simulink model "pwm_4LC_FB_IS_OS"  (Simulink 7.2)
settings: Solver=ode3  SolverMode=SingleTasking  StartTime=0.0  StopTime=0.1  FixedStep=10e-6  MaxStep=1e-4  RelTol=1e-3

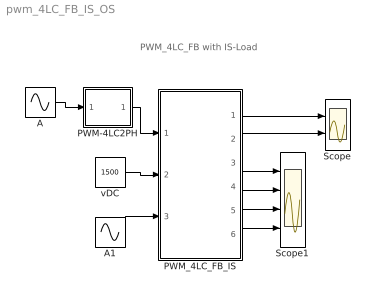
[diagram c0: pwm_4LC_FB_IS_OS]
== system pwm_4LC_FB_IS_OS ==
  note: PWM_4LC_FB with IS-Load
  A : Sin  Amplitude=.8  Frequency=2*pi*50  Phase=[0]  SampleTime=0
  A1 : Sin  Amplitude=500  Frequency=2*pi*50  Phase=[0 ]  SampleTime=0
  PWM-4LC2PH : Subsystem  mask(PWM-4LC1PH){FT=500, PHT1=0, PHT2=-120, PHT3=-240, DT=1e-6}
      mask prompts: FT "Frequency of Trian Sig."; PHT1 "Phase Angle of 1st Trian. Sig."; PHT2 "Phase Angle of 2nd Trian. Sig."; PHT3 "Phase Angle of 3rd Trian. Sig."; DT "Dead Time"
      mask help: Pulse Width Modulation for 1 Phase 4 Level Floating Capacitor Converter
  PWM_4LC_FB_IS : Subsystem  mask(pwm_4LC_FB_IS_OS){C1=10e-3, VC10=2*1500/3, C2=10e-3, VC20=1500/3}
      mask prompts: C1 "Cap C1"; VC10 "Initial Cap Voltage VC10"; C2 "Cap C2"; VC20 "Initial Cap Voltage VC20"
      mask help: Open Source 4-Level FC PWM FB Converter with IS load Input Vector u: u[0]= TD1.gate u[1]= TD2.gate u[2]= TD3.gate u[3]= TD4.gate u[4]= TD5.gate u[5]= TD6.gate u[6]= TD7.gate u[7]= TD8.gate u[8]= TD9.gate u[9]= TD10.gate u[10]= TD11.gate u[11]= TD12.gate u[12]= VDC u[13]= IA, Load Current as AC Current source Output Vector y: y[0]= Va.v, Output AC Voltage to middle point y[1]= Ia.I, Output AC Current y[2]= T1.I y[3]= D1.I y[4]= T1.V y[5]= T2.I y[6]= D2.I y[7]= T2.V y[8]= T3.I y[9]= D3.I y[10]= T3.V y[11]= IDC1, Input DC Current y[12]= IDC2, Input DC Current Parameter Vector p: p[0]= C1 p[1]= VC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
  Scope : Scope  NumInputPorts=2
  Scope1 : Scope  NumInputPorts=4
  vDC : Constant  Value=1500  OutDataType=sfix(16)  OutScaling=2^0
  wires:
  A/1 -> PWM-4LC2PH/1(In1)
  PWM-4LC2PH/1(Out1) -> PWM_4LC_FB_IS/1(Sw)
  PWM_4LC_FB_IS/1(vA) -> Scope/1
  PWM_4LC_FB_IS/2(iA) -> Scope/2
  vDC/1 -> PWM_4LC_FB_IS/2(vDC)
  A1/1 -> PWM_4LC_FB_IS/3(i_A)
  PWM_4LC_FB_IS/3(iT1,iD1,vT1) -> Scope1/1
  PWM_4LC_FB_IS/4(iT2,ID2,vT2) -> Scope1/2
  PWM_4LC_FB_IS/5(iT3,iD3,vT3) -> Scope1/3
  PWM_4LC_FB_IS/6(iDC1,IDC2) -> Scope1/4

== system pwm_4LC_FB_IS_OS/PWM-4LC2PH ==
  In1 : Inport  OutDataType=sfix(16)  OutScaling=2^0
  Gain : Gain  Gain=-1  ParameterDataType=sfix(16)  ParameterScaling=2^0  OutDataType=sfix(16)  OutScaling=2^0
  Mux : Mux  Inputs=2
  PWM-4LC1PH : Subsystem  mask(PWM-4LC1PH){FT=900, PHT1=0, PHT2=-120, PHT3=-240, DT=1e-6}
      mask prompts: FT "Frequency of Trian Sig."; PHT1 "Phase Angle of 1st Trian. Sig."; PHT2 "Phase Angle of 2nd Trian. Sig."; PHT3 "Phase Angle of 3rd Trian. Sig."; DT "Dead Time"
      mask help: Pulse Width Modulation for 1 Phase 4 Level Floating Capacitor Converter
  PWM-4LC1PH1 : Subsystem  mask(PWM-4LC1PH){FT=900, PHT1=0, PHT2=-120, PHT3=-240, DT=1e-6}
      mask prompts: FT "Frequency of Trian Sig."; PHT1 "Phase Angle of 1st Trian. Sig."; PHT2 "Phase Angle of 2nd Trian. Sig."; PHT3 "Phase Angle of 3rd Trian. Sig."; DT "Dead Time"
      mask help: Pulse Width Modulation for 1 Phase 4 Level Floating Capacitor Converter
  Out1 : Outport
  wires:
  In1/1 -> PWM-4LC1PH/1(In1), Gain/1
  PWM-4LC1PH1/1(Out1) -> Mux/2
  PWM-4LC1PH/1(Out1) -> Mux/1
  Mux/1 -> Out1/1
  Gain/1 -> PWM-4LC1PH1/1(In1)

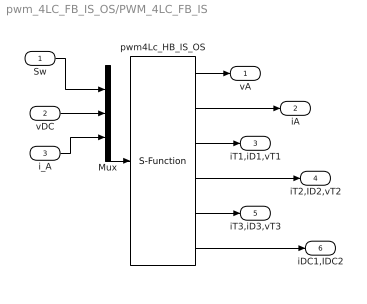
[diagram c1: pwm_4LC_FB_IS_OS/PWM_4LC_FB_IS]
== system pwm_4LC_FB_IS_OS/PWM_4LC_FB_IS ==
  Sw : Inport  OutDataType=sfix(16)  OutScaling=2^0
  vDC : Inport  Port=2  OutDataType=sfix(16)  OutScaling=2^0
  i_A : Inport  Port=3  OutDataType=sfix(16)  OutScaling=2^0
  Mux : Mux  Inputs="[12  1  1]"
  pwm4Lc_HB_IS_OS : S-Function  FunctionName=s_pwm_4LC_FB_IS_OS  Parameters="[C1  VC10  C2  VC20]"  EnableBusSupport=off
  vA : Outport  OutDataType=sfix(16)  OutScaling=2^0
  iA : Outport  Port=2  OutDataType=sfix(16)  OutScaling=2^0
  iT1,iD1,vT1 : Outport  Port=3  OutDataType=sfix(16)  OutScaling=2^0
  iT2,ID2,vT2 : Outport  Port=4  OutDataType=sfix(16)  OutScaling=2^0
  iT3,iD3,vT3 : Outport  Port=5  OutDataType=sfix(16)  OutScaling=2^0
  iDC1,IDC2 : Outport  Port=6  OutDataType=sfix(16)  OutScaling=2^0
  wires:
  pwm4Lc_HB_IS_OS/6 -> iDC1,IDC2/1
  pwm4Lc_HB_IS_OS/2 -> iA/1
  pwm4Lc_HB_IS_OS/1 -> vA/1
  i_A/1 -> Mux/3
  Mux/1 -> pwm4Lc_HB_IS_OS/1
  vDC/1 -> Mux/2
  Sw/1 -> Mux/1
  pwm4Lc_HB_IS_OS/3 -> iT1,iD1,vT1/1
  pwm4Lc_HB_IS_OS/4 -> iT2,ID2,vT2/1
  pwm4Lc_HB_IS_OS/5 -> iT3,iD3,vT3/1

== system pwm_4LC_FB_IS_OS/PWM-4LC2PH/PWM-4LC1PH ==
  In1 : Inport  OutDataType=sfix(16)  OutScaling=2^0
  Mux : Mux  Inputs=6
  PWM-2L-1PH : Subsystem  mask(PWM-2L-1PH){FT=FT, PHT=PHT1, DT=DT}
      mask prompts: FT "Triangular Frequency"; PHT "Trian. Phase Angle (Degree)"; DT "Dead Time"
      mask help: Pulse Width Modulation for 1 Phase Converter
  PWM-2L-1PH1 : Subsystem  mask(PWM-2L-1PH){FT=FT, PHT=PHT2, DT=DT}
      mask prompts: FT "Triangular Frequency"; PHT "Trian. Phase Angle (Degree)"; DT "Dead Time"
      mask help: Pulse Width Modulation for 1 Phase Converter
  PWM-2L-1PH2 : Subsystem  mask(PWM-2L-1PH){FT=FT, PHT=PHT3, DT=DT}
      mask prompts: FT "Triangular Frequency"; PHT "Trian. Phase Angle (Degree)"; DT "Dead Time"
      mask help: Pulse Width Modulation for 1 Phase Converter
  Out1 : Outport
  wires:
  PWM-2L-1PH/1(Out1) -> Mux/1
  PWM-2L-1PH1/1(Out1) -> Mux/2
  PWM-2L-1PH1/2(Out2) -> Mux/5
  PWM-2L-1PH2/1(Out1) -> Mux/3
  PWM-2L-1PH2/2(Out2) -> Mux/4
  Mux/1 -> Out1/1
  In1/1 -> PWM-2L-1PH/1(In1), PWM-2L-1PH1/1(In1), PWM-2L-1PH2/1(In1)
  PWM-2L-1PH/2(Out2) -> Mux/6

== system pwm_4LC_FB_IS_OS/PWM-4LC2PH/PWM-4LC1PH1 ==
  In1 : Inport  OutDataType=sfix(16)  OutScaling=2^0
  Mux : Mux  Inputs=6
  PWM-2L-1PH : Subsystem  mask(PWM-2L-1PH){FT=FT, PHT=PHT1, DT=DT}
      mask prompts: FT "Triangular Frequency"; PHT "Trian. Phase Angle (Degree)"; DT "Dead Time"
      mask help: Pulse Width Modulation for 1 Phase Converter
  PWM-2L-1PH1 : Subsystem  mask(PWM-2L-1PH){FT=FT, PHT=PHT2, DT=DT}
      mask prompts: FT "Triangular Frequency"; PHT "Trian. Phase Angle (Degree)"; DT "Dead Time"
      mask help: Pulse Width Modulation for 1 Phase Converter
  PWM-2L-1PH2 : Subsystem  mask(PWM-2L-1PH){FT=FT, PHT=PHT3, DT=DT}
      mask prompts: FT "Triangular Frequency"; PHT "Trian. Phase Angle (Degree)"; DT "Dead Time"
      mask help: Pulse Width Modulation for 1 Phase Converter
  Out1 : Outport
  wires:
  PWM-2L-1PH/2(Out2) -> Mux/6
  In1/1 -> PWM-2L-1PH2/1(In1), PWM-2L-1PH1/1(In1), PWM-2L-1PH/1(In1)
  Mux/1 -> Out1/1
  PWM-2L-1PH2/2(Out2) -> Mux/4
  PWM-2L-1PH2/1(Out1) -> Mux/3
  PWM-2L-1PH1/2(Out2) -> Mux/5
  PWM-2L-1PH1/1(Out1) -> Mux/2
  PWM-2L-1PH/1(Out1) -> Mux/1

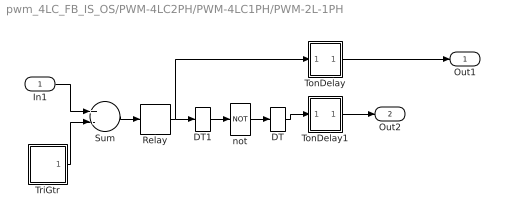
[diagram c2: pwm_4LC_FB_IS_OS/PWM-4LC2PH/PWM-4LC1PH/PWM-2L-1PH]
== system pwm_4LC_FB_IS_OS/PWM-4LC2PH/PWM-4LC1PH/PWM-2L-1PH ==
  In1 : Inport  OutDataType=sfix(16)  OutScaling=2^0
  DT : DataTypeConversion
  DT1 : DataTypeConversion
  Relay : Relay  OutDataType=sfix(16)  OutScaling=2^0
  Sum : Sum  Inputs=+-  OutDataType=sfix(16)  OutScaling=2^0
  TonDelay : Subsystem  mask(TonDelay){DT=DT}
      mask prompts: DT "Dead Time"
      mask help: Turn on dead time to protect against short circuit of the converter leg
  TonDelay1 : Subsystem  mask(TonDelay){DT=DT}
      mask prompts: DT "Dead Time"
      mask help: Turn on dead time to protect against short circuit of the converter leg
  TriGtr : Subsystem  mask(TriGtr){T=1/FT, Td=PHT/FT/360}
      mask prompts: T "Period Time"; Td "Time Delay"
      mask help: Triangular Wave Generator with variable time delay
  not : Logic  Operator=NOT  Inputs=1
  Out1 : Outport  InitialOutput=0
  Out2 : Outport  Port=2  InitialOutput=0
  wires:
  DT1/1 -> not/1
  DT/1 -> TonDelay1/1(s1)
  In1/1 -> Sum/1
  TriGtr/1(O) -> Sum/2
  Sum/1 -> Relay/1
  not/1 -> DT/1
  TonDelay1/1(s1d) -> Out2/1
  Relay/1 -> DT1/1, TonDelay/1(s1)
  TonDelay/1(s1d) -> Out1/1

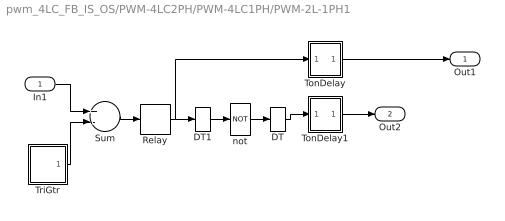
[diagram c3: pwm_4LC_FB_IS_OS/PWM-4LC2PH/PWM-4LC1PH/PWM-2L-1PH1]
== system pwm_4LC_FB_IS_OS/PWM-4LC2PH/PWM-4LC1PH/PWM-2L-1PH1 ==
  In1 : Inport  OutDataType=sfix(16)  OutScaling=2^0
  DT : DataTypeConversion
  DT1 : DataTypeConversion
  Relay : Relay  OutDataType=sfix(16)  OutScaling=2^0
  Sum : Sum  Inputs=+-  OutDataType=sfix(16)  OutScaling=2^0
  TonDelay : Subsystem  mask(TonDelay){DT=DT}
      mask prompts: DT "Dead Time"
      mask help: Turn on dead time to protect against short circuit of the converter leg
  TonDelay1 : Subsystem  mask(TonDelay){DT=DT}
      mask prompts: DT "Dead Time"
      mask help: Turn on dead time to protect against short circuit of the converter leg
  TriGtr : Subsystem  mask(TriGtr){T=1/FT, Td=PHT/FT/360}
      mask prompts: T "Period Time"; Td "Time Delay"
      mask help: Triangular Wave Generator with variable time delay
  not : Logic  Operator=NOT  Inputs=1
  Out1 : Outport  InitialOutput=0
  Out2 : Outport  Port=2  InitialOutput=0
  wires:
  TonDelay/1(s1d) -> Out1/1
  Relay/1 -> TonDelay/1(s1), DT1/1
  TonDelay1/1(s1d) -> Out2/1
  not/1 -> DT/1
  Sum/1 -> Relay/1
  TriGtr/1(O) -> Sum/2
  In1/1 -> Sum/1
  DT/1 -> TonDelay1/1(s1)
  DT1/1 -> not/1

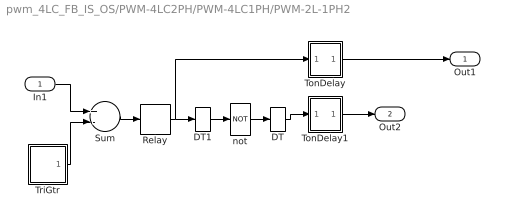
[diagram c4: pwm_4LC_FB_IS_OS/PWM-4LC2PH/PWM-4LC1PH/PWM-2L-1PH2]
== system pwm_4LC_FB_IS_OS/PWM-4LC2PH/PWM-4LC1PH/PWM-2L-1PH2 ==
  In1 : Inport  OutDataType=sfix(16)  OutScaling=2^0
  DT : DataTypeConversion
  DT1 : DataTypeConversion
  Relay : Relay  OutDataType=sfix(16)  OutScaling=2^0
  Sum : Sum  Inputs=+-  OutDataType=sfix(16)  OutScaling=2^0
  TonDelay : Subsystem  mask(TonDelay){DT=DT}
      mask prompts: DT "Dead Time"
      mask help: Turn on dead time to protect against short circuit of the converter leg
  TonDelay1 : Subsystem  mask(TonDelay){DT=DT}
      mask prompts: DT "Dead Time"
      mask help: Turn on dead time to protect against short circuit of the converter leg
  TriGtr : Subsystem  mask(TriGtr){T=1/FT, Td=PHT/FT/360}
      mask prompts: T "Period Time"; Td "Time Delay"
      mask help: Triangular Wave Generator with variable time delay
  not : Logic  Operator=NOT  Inputs=1
  Out1 : Outport  InitialOutput=0
  Out2 : Outport  Port=2  InitialOutput=0
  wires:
  DT1/1 -> not/1
  DT/1 -> TonDelay1/1(s1)
  In1/1 -> Sum/1
  TriGtr/1(O) -> Sum/2
  Sum/1 -> Relay/1
  not/1 -> DT/1
  TonDelay1/1(s1d) -> Out2/1
  Relay/1 -> DT1/1, TonDelay/1(s1)
  TonDelay/1(s1d) -> Out1/1

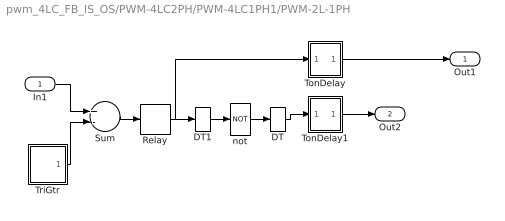
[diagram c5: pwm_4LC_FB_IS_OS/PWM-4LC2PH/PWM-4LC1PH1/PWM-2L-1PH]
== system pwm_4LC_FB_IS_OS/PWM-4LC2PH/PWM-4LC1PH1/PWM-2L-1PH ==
  In1 : Inport  OutDataType=sfix(16)  OutScaling=2^0
  DT : DataTypeConversion
  DT1 : DataTypeConversion
  Relay : Relay  OutDataType=sfix(16)  OutScaling=2^0
  Sum : Sum  Inputs=+-  OutDataType=sfix(16)  OutScaling=2^0
  TonDelay : Subsystem  mask(TonDelay){DT=DT}
      mask prompts: DT "Dead Time"
      mask help: Turn on dead time to protect against short circuit of the converter leg
  TonDelay1 : Subsystem  mask(TonDelay){DT=DT}
      mask prompts: DT "Dead Time"
      mask help: Turn on dead time to protect against short circuit of the converter leg
  TriGtr : Subsystem  mask(TriGtr){T=1/FT, Td=PHT/FT/360}
      mask prompts: T "Period Time"; Td "Time Delay"
      mask help: Triangular Wave Generator with variable time delay
  not : Logic  Operator=NOT  Inputs=1
  Out1 : Outport  InitialOutput=0
  Out2 : Outport  Port=2  InitialOutput=0
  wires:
  TonDelay/1(s1d) -> Out1/1
  Relay/1 -> TonDelay/1(s1), DT1/1
  TonDelay1/1(s1d) -> Out2/1
  not/1 -> DT/1
  Sum/1 -> Relay/1
  TriGtr/1(O) -> Sum/2
  In1/1 -> Sum/1
  DT/1 -> TonDelay1/1(s1)
  DT1/1 -> not/1

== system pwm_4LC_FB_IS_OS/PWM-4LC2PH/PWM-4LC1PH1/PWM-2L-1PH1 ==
  In1 : Inport  OutDataType=sfix(16)  OutScaling=2^0
  DT : DataTypeConversion
  DT1 : DataTypeConversion
  Relay : Relay  OutDataType=sfix(16)  OutScaling=2^0
  Sum : Sum  Inputs=+-  OutDataType=sfix(16)  OutScaling=2^0
  TonDelay : Subsystem  mask(TonDelay){DT=DT}
      mask prompts: DT "Dead Time"
      mask help: Turn on dead time to protect against short circuit of the converter leg
  TonDelay1 : Subsystem  mask(TonDelay){DT=DT}
      mask prompts: DT "Dead Time"
      mask help: Turn on dead time to protect against short circuit of the converter leg
  TriGtr : Subsystem  mask(TriGtr){T=1/FT, Td=PHT/FT/360}
      mask prompts: T "Period Time"; Td "Time Delay"
      mask help: Triangular Wave Generator with variable time delay
  not : Logic  Operator=NOT  Inputs=1
  Out1 : Outport  InitialOutput=0
  Out2 : Outport  Port=2  InitialOutput=0
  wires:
  DT1/1 -> not/1
  DT/1 -> TonDelay1/1(s1)
  In1/1 -> Sum/1
  TriGtr/1(O) -> Sum/2
  Sum/1 -> Relay/1
  not/1 -> DT/1
  TonDelay1/1(s1d) -> Out2/1
  Relay/1 -> DT1/1, TonDelay/1(s1)
  TonDelay/1(s1d) -> Out1/1

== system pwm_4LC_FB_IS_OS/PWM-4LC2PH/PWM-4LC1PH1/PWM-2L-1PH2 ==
  In1 : Inport  OutDataType=sfix(16)  OutScaling=2^0
  DT : DataTypeConversion
  DT1 : DataTypeConversion
  Relay : Relay  OutDataType=sfix(16)  OutScaling=2^0
  Sum : Sum  Inputs=+-  OutDataType=sfix(16)  OutScaling=2^0
  TonDelay : Subsystem  mask(TonDelay){DT=DT}
      mask prompts: DT "Dead Time"
      mask help: Turn on dead time to protect against short circuit of the converter leg
  TonDelay1 : Subsystem  mask(TonDelay){DT=DT}
      mask prompts: DT "Dead Time"
      mask help: Turn on dead time to protect against short circuit of the converter leg
  TriGtr : Subsystem  mask(TriGtr){T=1/FT, Td=PHT/FT/360}
      mask prompts: T "Period Time"; Td "Time Delay"
      mask help: Triangular Wave Generator with variable time delay
  not : Logic  Operator=NOT  Inputs=1
  Out1 : Outport  InitialOutput=0
  Out2 : Outport  Port=2  InitialOutput=0
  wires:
  TonDelay/1(s1d) -> Out1/1
  Relay/1 -> TonDelay/1(s1), DT1/1
  TonDelay1/1(s1d) -> Out2/1
  not/1 -> DT/1
  Sum/1 -> Relay/1
  TriGtr/1(O) -> Sum/2
  In1/1 -> Sum/1
  DT/1 -> TonDelay1/1(s1)
  DT1/1 -> not/1

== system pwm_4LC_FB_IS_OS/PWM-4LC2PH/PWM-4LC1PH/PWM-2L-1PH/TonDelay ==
  s1 : Inport  Orientation=down  OutDataType=sfix(16)  OutScaling=2^0
  Int : Integrator  ExternalReset=falling
  Rel1 : Relay  OnSwitchValue=DT  OutDataType=sfix(16)  OutScaling=2^0
  s1d : Outport  InitialOutput=0
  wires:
  Int/1 -> Rel1/1
  s1/1 -> Int/2, Int/1
  Rel1/1 -> s1d/1

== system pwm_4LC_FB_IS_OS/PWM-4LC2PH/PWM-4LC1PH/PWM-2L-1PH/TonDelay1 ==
  s1 : Inport  Orientation=down  OutDataType=sfix(16)  OutScaling=2^0
  Int : Integrator  ExternalReset=falling
  Rel1 : Relay  OnSwitchValue=DT  OutDataType=sfix(16)  OutScaling=2^0
  s1d : Outport  InitialOutput=0
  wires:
  Int/1 -> Rel1/1
  s1/1 -> Int/2, Int/1
  Rel1/1 -> s1d/1

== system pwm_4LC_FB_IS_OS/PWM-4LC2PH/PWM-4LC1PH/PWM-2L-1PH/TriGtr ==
  Clock : Clock
  S1 : Subsystem
  Sum : Sum  OutDataType=sfix(16)  OutScaling=2^0
  T : Constant  Value=T  OutDataType=sfix(16)  OutScaling=2^0
  Td : Constant  Value=Td  OutDataType=sfix(16)  OutScaling=2^0
  mod : Math  Operator=mod
  O : Outport  InitialOutput=0
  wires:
  mod/1 -> S1/1(In1)
  S1/1(Out1) -> O/1
  Clock/1 -> Sum/1
  T/1 -> mod/2
  Sum/1 -> mod/1
  Td/1 -> Sum/2

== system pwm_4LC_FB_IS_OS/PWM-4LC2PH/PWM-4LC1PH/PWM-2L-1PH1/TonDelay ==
  s1 : Inport  Orientation=down  OutDataType=sfix(16)  OutScaling=2^0
  Int : Integrator  ExternalReset=falling
  Rel1 : Relay  OnSwitchValue=DT  OutDataType=sfix(16)  OutScaling=2^0
  s1d : Outport  InitialOutput=0
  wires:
  Rel1/1 -> s1d/1
  s1/1 -> Int/1, Int/2
  Int/1 -> Rel1/1

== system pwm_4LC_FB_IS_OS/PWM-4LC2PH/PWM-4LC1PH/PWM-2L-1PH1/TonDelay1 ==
  s1 : Inport  Orientation=down  OutDataType=sfix(16)  OutScaling=2^0
  Int : Integrator  ExternalReset=falling
  Rel1 : Relay  OnSwitchValue=DT  OutDataType=sfix(16)  OutScaling=2^0
  s1d : Outport  InitialOutput=0
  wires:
  Rel1/1 -> s1d/1
  s1/1 -> Int/1, Int/2
  Int/1 -> Rel1/1

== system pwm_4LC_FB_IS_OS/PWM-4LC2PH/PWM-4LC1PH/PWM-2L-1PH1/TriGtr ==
  Clock : Clock
  S1 : Subsystem
  Sum : Sum  OutDataType=sfix(16)  OutScaling=2^0
  T : Constant  Value=T  OutDataType=sfix(16)  OutScaling=2^0
  Td : Constant  Value=Td  OutDataType=sfix(16)  OutScaling=2^0
  mod : Math  Operator=mod
  O : Outport  InitialOutput=0
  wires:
  Td/1 -> Sum/2
  Sum/1 -> mod/1
  T/1 -> mod/2
  Clock/1 -> Sum/1
  S1/1(Out1) -> O/1
  mod/1 -> S1/1(In1)

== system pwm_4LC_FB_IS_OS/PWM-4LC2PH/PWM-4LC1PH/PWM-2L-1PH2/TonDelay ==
  s1 : Inport  Orientation=down  OutDataType=sfix(16)  OutScaling=2^0
  Int : Integrator  ExternalReset=falling
  Rel1 : Relay  OnSwitchValue=DT  OutDataType=sfix(16)  OutScaling=2^0
  s1d : Outport  InitialOutput=0
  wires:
  Int/1 -> Rel1/1
  s1/1 -> Int/2, Int/1
  Rel1/1 -> s1d/1

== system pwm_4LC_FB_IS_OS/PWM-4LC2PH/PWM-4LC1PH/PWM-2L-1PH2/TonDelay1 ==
  s1 : Inport  Orientation=down  OutDataType=sfix(16)  OutScaling=2^0
  Int : Integrator  ExternalReset=falling
  Rel1 : Relay  OnSwitchValue=DT  OutDataType=sfix(16)  OutScaling=2^0
  s1d : Outport  InitialOutput=0
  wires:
  Int/1 -> Rel1/1
  s1/1 -> Int/2, Int/1
  Rel1/1 -> s1d/1

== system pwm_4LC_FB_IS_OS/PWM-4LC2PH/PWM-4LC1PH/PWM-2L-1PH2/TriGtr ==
  Clock : Clock
  S1 : Subsystem
  Sum : Sum  OutDataType=sfix(16)  OutScaling=2^0
  T : Constant  Value=T  OutDataType=sfix(16)  OutScaling=2^0
  Td : Constant  Value=Td  OutDataType=sfix(16)  OutScaling=2^0
  mod : Math  Operator=mod
  O : Outport  InitialOutput=0
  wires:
  mod/1 -> S1/1(In1)
  S1/1(Out1) -> O/1
  Clock/1 -> Sum/1
  T/1 -> mod/2
  Sum/1 -> mod/1
  Td/1 -> Sum/2

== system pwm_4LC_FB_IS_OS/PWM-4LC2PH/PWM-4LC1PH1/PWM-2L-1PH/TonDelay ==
  s1 : Inport  Orientation=down  OutDataType=sfix(16)  OutScaling=2^0
  Int : Integrator  ExternalReset=falling
  Rel1 : Relay  OnSwitchValue=DT  OutDataType=sfix(16)  OutScaling=2^0
  s1d : Outport  InitialOutput=0
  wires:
  Rel1/1 -> s1d/1
  s1/1 -> Int/1, Int/2
  Int/1 -> Rel1/1

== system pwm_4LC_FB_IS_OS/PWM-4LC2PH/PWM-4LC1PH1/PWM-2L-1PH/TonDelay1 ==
  s1 : Inport  Orientation=down  OutDataType=sfix(16)  OutScaling=2^0
  Int : Integrator  ExternalReset=falling
  Rel1 : Relay  OnSwitchValue=DT  OutDataType=sfix(16)  OutScaling=2^0
  s1d : Outport  InitialOutput=0
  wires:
  Rel1/1 -> s1d/1
  s1/1 -> Int/1, Int/2
  Int/1 -> Rel1/1

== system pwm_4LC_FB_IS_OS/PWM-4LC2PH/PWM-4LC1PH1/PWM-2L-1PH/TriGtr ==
  Clock : Clock
  S1 : Subsystem
  Sum : Sum  OutDataType=sfix(16)  OutScaling=2^0
  T : Constant  Value=T  OutDataType=sfix(16)  OutScaling=2^0
  Td : Constant  Value=Td  OutDataType=sfix(16)  OutScaling=2^0
  mod : Math  Operator=mod
  O : Outport  InitialOutput=0
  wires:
  Td/1 -> Sum/2
  Sum/1 -> mod/1
  T/1 -> mod/2
  Clock/1 -> Sum/1
  S1/1(Out1) -> O/1
  mod/1 -> S1/1(In1)

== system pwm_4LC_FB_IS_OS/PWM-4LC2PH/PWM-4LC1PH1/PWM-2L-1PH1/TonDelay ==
  s1 : Inport  Orientation=down  OutDataType=sfix(16)  OutScaling=2^0
  Int : Integrator  ExternalReset=falling
  Rel1 : Relay  OnSwitchValue=DT  OutDataType=sfix(16)  OutScaling=2^0
  s1d : Outport  InitialOutput=0
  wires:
  Int/1 -> Rel1/1
  s1/1 -> Int/2, Int/1
  Rel1/1 -> s1d/1

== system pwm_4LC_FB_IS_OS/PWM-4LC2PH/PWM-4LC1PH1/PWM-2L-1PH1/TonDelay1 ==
  s1 : Inport  Orientation=down  OutDataType=sfix(16)  OutScaling=2^0
  Int : Integrator  ExternalReset=falling
  Rel1 : Relay  OnSwitchValue=DT  OutDataType=sfix(16)  OutScaling=2^0
  s1d : Outport  InitialOutput=0
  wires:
  Int/1 -> Rel1/1
  s1/1 -> Int/2, Int/1
  Rel1/1 -> s1d/1

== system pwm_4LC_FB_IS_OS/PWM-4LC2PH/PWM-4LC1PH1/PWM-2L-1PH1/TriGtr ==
  Clock : Clock
  S1 : Subsystem
  Sum : Sum  OutDataType=sfix(16)  OutScaling=2^0
  T : Constant  Value=T  OutDataType=sfix(16)  OutScaling=2^0
  Td : Constant  Value=Td  OutDataType=sfix(16)  OutScaling=2^0
  mod : Math  Operator=mod
  O : Outport  InitialOutput=0
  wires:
  mod/1 -> S1/1(In1)
  S1/1(Out1) -> O/1
  Clock/1 -> Sum/1
  T/1 -> mod/2
  Sum/1 -> mod/1
  Td/1 -> Sum/2

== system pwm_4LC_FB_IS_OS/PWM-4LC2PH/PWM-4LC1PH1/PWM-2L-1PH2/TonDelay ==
  s1 : Inport  Orientation=down  OutDataType=sfix(16)  OutScaling=2^0
  Int : Integrator  ExternalReset=falling
  Rel1 : Relay  OnSwitchValue=DT  OutDataType=sfix(16)  OutScaling=2^0
  s1d : Outport  InitialOutput=0
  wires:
  Rel1/1 -> s1d/1
  s1/1 -> Int/1, Int/2
  Int/1 -> Rel1/1

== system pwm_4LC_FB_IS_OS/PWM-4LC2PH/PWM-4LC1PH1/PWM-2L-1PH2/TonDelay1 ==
  s1 : Inport  Orientation=down  OutDataType=sfix(16)  OutScaling=2^0
  Int : Integrator  ExternalReset=falling
  Rel1 : Relay  OnSwitchValue=DT  OutDataType=sfix(16)  OutScaling=2^0
  s1d : Outport  InitialOutput=0
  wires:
  Rel1/1 -> s1d/1
  s1/1 -> Int/1, Int/2
  Int/1 -> Rel1/1

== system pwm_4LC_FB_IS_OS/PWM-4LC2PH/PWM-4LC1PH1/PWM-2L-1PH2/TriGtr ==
  Clock : Clock
  S1 : Subsystem
  Sum : Sum  OutDataType=sfix(16)  OutScaling=2^0
  T : Constant  Value=T  OutDataType=sfix(16)  OutScaling=2^0
  Td : Constant  Value=Td  OutDataType=sfix(16)  OutScaling=2^0
  mod : Math  Operator=mod
  O : Outport  InitialOutput=0
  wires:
  Td/1 -> Sum/2
  Sum/1 -> mod/1
  T/1 -> mod/2
  Clock/1 -> Sum/1
  S1/1(Out1) -> O/1
  mod/1 -> S1/1(In1)

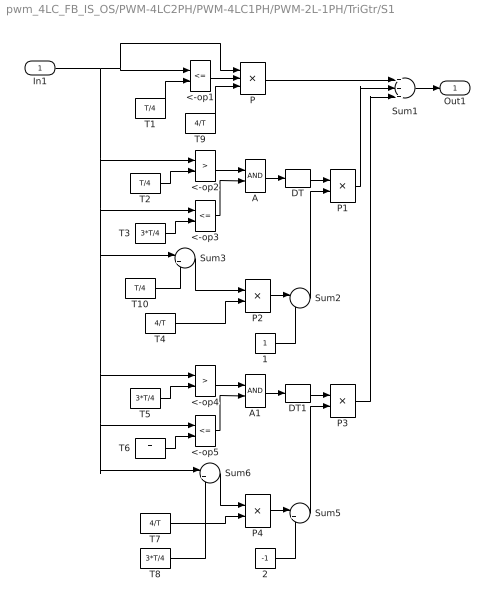
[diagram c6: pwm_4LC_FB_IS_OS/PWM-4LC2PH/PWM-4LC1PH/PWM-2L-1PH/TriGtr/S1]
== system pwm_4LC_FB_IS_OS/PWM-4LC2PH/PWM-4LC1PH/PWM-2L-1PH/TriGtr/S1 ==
  In1 : Inport  OutDataType=sfix(16)  OutScaling=2^0
  1 : Constant  OutDataType=sfix(16)  OutScaling=2^0
  2 : Constant  Value=-1  OutDataType=sfix(16)  OutScaling=2^0
  <-op1 : RelationalOperator  Operator=<=
  <-op2 : RelationalOperator  Operator=>
  <-op3 : RelationalOperator  Operator=<=
  <-op4 : RelationalOperator  Operator=>
  <-op5 : RelationalOperator  Operator=<=
  A : Logic  AllPortsSameDT=off
  A1 : Logic  AllPortsSameDT=off
  DT : DataTypeConversion
  DT1 : DataTypeConversion
  P : Product  Inputs=3  OutDataType=sfix(16)  OutScaling=2^0
  P{1..4} (4 alike) : Product  OutDataType=sfix(16)  OutScaling=2^0
  Sum1 : Sum  Inputs=+++  OutDataType=sfix(16)  OutScaling=2^0
  Sum2 : Sum  Inputs=|-+  OutDataType=sfix(16)  OutScaling=2^0
  Sum3 : Sum  Inputs=|+-  OutDataType=sfix(16)  OutScaling=2^0
  Sum5 : Sum  Inputs=|++  OutDataType=sfix(16)  OutScaling=2^0
  Sum6 : Sum  Inputs=|+-  OutDataType=sfix(16)  OutScaling=2^0
  T1 : Constant  Value=T/4  OutDataType=sfix(16)  OutScaling=2^0
  T10 : Constant  Value=T/4  OutDataType=sfix(16)  OutScaling=2^0
  T2 : Constant  Value=T/4  OutDataType=sfix(16)  OutScaling=2^0
  T3 : Constant  Value=3*T/4  OutDataType=sfix(16)  OutScaling=2^0
  T4 : Constant  Value=4/T  OutDataType=sfix(16)  OutScaling=2^0
  T5 : Constant  Value=3*T/4  OutDataType=sfix(16)  OutScaling=2^0
  T6 : Constant  Value=T  OutDataType=sfix(16)  OutScaling=2^0
  T7 : Constant  Value=4/T  OutDataType=sfix(16)  OutScaling=2^0
  T8 : Constant  Value=3*T/4  OutDataType=sfix(16)  OutScaling=2^0
  T9 : Constant  Value=4/T  OutDataType=sfix(16)  OutScaling=2^0
  Out1 : Outport
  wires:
  Sum1/1 -> Out1/1
  P3/1 -> Sum1/3
  T8/1 -> Sum6/2
  Sum5/1 -> P3/2
  2/1 -> Sum5/2
  P4/1 -> Sum5/1
  Sum6/1 -> P4/1
  T7/1 -> P4/2
  A1/1 -> DT1/1
  <-op5/1 -> A1/2
  T6/1 -> <-op5/2
  <-op4/1 -> A1/1
  T5/1 -> <-op4/2
  Sum2/1 -> P1/2
  1/1 -> Sum2/2
  P2/1 -> Sum2/1
  P1/1 -> Sum1/2
  In1/1 -> P/1, <-op1/1, Sum6/1, <-op5/1, <-op4/1, Sum3/1, <-op3/1, <-op2/1
  Sum3/1 -> P2/1
  T4/1 -> P2/2
  A/1 -> DT/1
  <-op3/1 -> A/2
  T3/1 -> <-op3/2
  <-op2/1 -> A/1
  T2/1 -> <-op2/2
  P/1 -> Sum1/1
  <-op1/1 -> P/2
  T1/1 -> <-op1/2
  DT/1 -> P1/1
  DT1/1 -> P3/1
  T9/1 -> P/3
  T10/1 -> Sum3/2

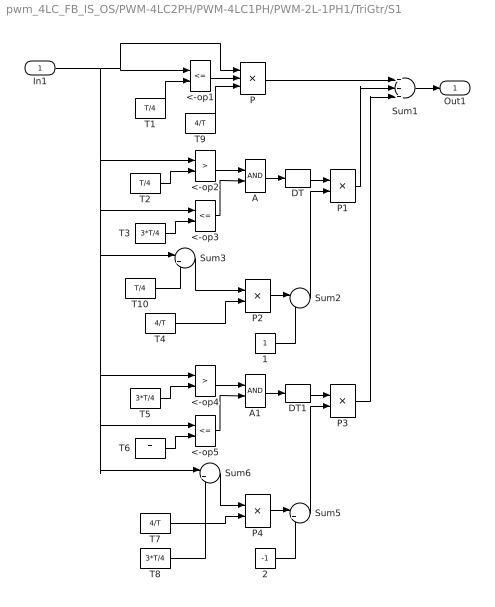
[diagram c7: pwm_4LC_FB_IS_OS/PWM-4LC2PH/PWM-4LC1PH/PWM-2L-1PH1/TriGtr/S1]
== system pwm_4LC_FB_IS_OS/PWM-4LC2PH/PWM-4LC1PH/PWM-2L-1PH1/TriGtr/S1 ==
  In1 : Inport  OutDataType=sfix(16)  OutScaling=2^0
  1 : Constant  OutDataType=sfix(16)  OutScaling=2^0
  2 : Constant  Value=-1  OutDataType=sfix(16)  OutScaling=2^0
  <-op1 : RelationalOperator  Operator=<=
  <-op2 : RelationalOperator  Operator=>
  <-op3 : RelationalOperator  Operator=<=
  <-op4 : RelationalOperator  Operator=>
  <-op5 : RelationalOperator  Operator=<=
  A : Logic  AllPortsSameDT=off
  A1 : Logic  AllPortsSameDT=off
  DT : DataTypeConversion
  DT1 : DataTypeConversion
  P : Product  Inputs=3  OutDataType=sfix(16)  OutScaling=2^0
  P{1..4} (4 alike) : Product  OutDataType=sfix(16)  OutScaling=2^0
  Sum1 : Sum  Inputs=+++  OutDataType=sfix(16)  OutScaling=2^0
  Sum2 : Sum  Inputs=|-+  OutDataType=sfix(16)  OutScaling=2^0
  Sum3 : Sum  Inputs=|+-  OutDataType=sfix(16)  OutScaling=2^0
  Sum5 : Sum  Inputs=|++  OutDataType=sfix(16)  OutScaling=2^0
  Sum6 : Sum  Inputs=|+-  OutDataType=sfix(16)  OutScaling=2^0
  T1 : Constant  Value=T/4  OutDataType=sfix(16)  OutScaling=2^0
  T10 : Constant  Value=T/4  OutDataType=sfix(16)  OutScaling=2^0
  T2 : Constant  Value=T/4  OutDataType=sfix(16)  OutScaling=2^0
  T3 : Constant  Value=3*T/4  OutDataType=sfix(16)  OutScaling=2^0
  T4 : Constant  Value=4/T  OutDataType=sfix(16)  OutScaling=2^0
  T5 : Constant  Value=3*T/4  OutDataType=sfix(16)  OutScaling=2^0
  T6 : Constant  Value=T  OutDataType=sfix(16)  OutScaling=2^0
  T7 : Constant  Value=4/T  OutDataType=sfix(16)  OutScaling=2^0
  T8 : Constant  Value=3*T/4  OutDataType=sfix(16)  OutScaling=2^0
  T9 : Constant  Value=4/T  OutDataType=sfix(16)  OutScaling=2^0
  Out1 : Outport
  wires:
  T10/1 -> Sum3/2
  T9/1 -> P/3
  DT1/1 -> P3/1
  DT/1 -> P1/1
  T1/1 -> <-op1/2
  <-op1/1 -> P/2
  P/1 -> Sum1/1
  T2/1 -> <-op2/2
  <-op2/1 -> A/1
  T3/1 -> <-op3/2
  <-op3/1 -> A/2
  A/1 -> DT/1
  T4/1 -> P2/2
  Sum3/1 -> P2/1
  In1/1 -> <-op2/1, <-op3/1, Sum3/1, <-op4/1, <-op5/1, Sum6/1, <-op1/1, P/1
  P1/1 -> Sum1/2
  P2/1 -> Sum2/1
  1/1 -> Sum2/2
  Sum2/1 -> P1/2
  T5/1 -> <-op4/2
  <-op4/1 -> A1/1
  T6/1 -> <-op5/2
  <-op5/1 -> A1/2
  A1/1 -> DT1/1
  T7/1 -> P4/2
  Sum6/1 -> P4/1
  P4/1 -> Sum5/1
  2/1 -> Sum5/2
  Sum5/1 -> P3/2
  T8/1 -> Sum6/2
  P3/1 -> Sum1/3
  Sum1/1 -> Out1/1

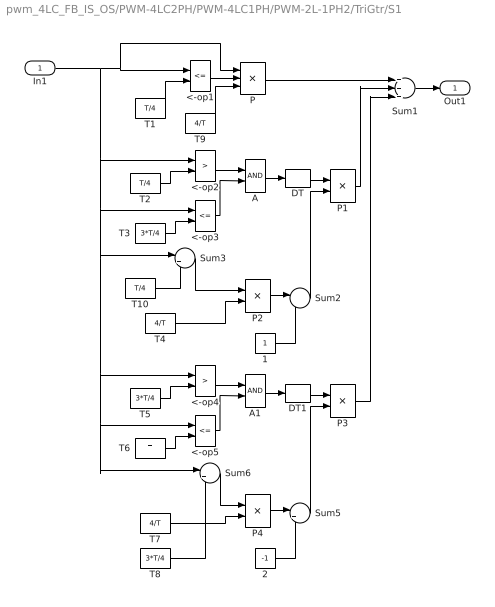
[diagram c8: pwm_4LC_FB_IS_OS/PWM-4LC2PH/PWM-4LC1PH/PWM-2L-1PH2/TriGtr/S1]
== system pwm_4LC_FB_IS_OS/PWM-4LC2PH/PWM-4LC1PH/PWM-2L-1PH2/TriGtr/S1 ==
  In1 : Inport  OutDataType=sfix(16)  OutScaling=2^0
  1 : Constant  OutDataType=sfix(16)  OutScaling=2^0
  2 : Constant  Value=-1  OutDataType=sfix(16)  OutScaling=2^0
  <-op1 : RelationalOperator  Operator=<=
  <-op2 : RelationalOperator  Operator=>
  <-op3 : RelationalOperator  Operator=<=
  <-op4 : RelationalOperator  Operator=>
  <-op5 : RelationalOperator  Operator=<=
  A : Logic  AllPortsSameDT=off
  A1 : Logic  AllPortsSameDT=off
  DT : DataTypeConversion
  DT1 : DataTypeConversion
  P : Product  Inputs=3  OutDataType=sfix(16)  OutScaling=2^0
  P{1..4} (4 alike) : Product  OutDataType=sfix(16)  OutScaling=2^0
  Sum1 : Sum  Inputs=+++  OutDataType=sfix(16)  OutScaling=2^0
  Sum2 : Sum  Inputs=|-+  OutDataType=sfix(16)  OutScaling=2^0
  Sum3 : Sum  Inputs=|+-  OutDataType=sfix(16)  OutScaling=2^0
  Sum5 : Sum  Inputs=|++  OutDataType=sfix(16)  OutScaling=2^0
  Sum6 : Sum  Inputs=|+-  OutDataType=sfix(16)  OutScaling=2^0
  T1 : Constant  Value=T/4  OutDataType=sfix(16)  OutScaling=2^0
  T10 : Constant  Value=T/4  OutDataType=sfix(16)  OutScaling=2^0
  T2 : Constant  Value=T/4  OutDataType=sfix(16)  OutScaling=2^0
  T3 : Constant  Value=3*T/4  OutDataType=sfix(16)  OutScaling=2^0
  T4 : Constant  Value=4/T  OutDataType=sfix(16)  OutScaling=2^0
  T5 : Constant  Value=3*T/4  OutDataType=sfix(16)  OutScaling=2^0
  T6 : Constant  Value=T  OutDataType=sfix(16)  OutScaling=2^0
  T7 : Constant  Value=4/T  OutDataType=sfix(16)  OutScaling=2^0
  T8 : Constant  Value=3*T/4  OutDataType=sfix(16)  OutScaling=2^0
  T9 : Constant  Value=4/T  OutDataType=sfix(16)  OutScaling=2^0
  Out1 : Outport
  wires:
  Sum1/1 -> Out1/1
  P3/1 -> Sum1/3
  T8/1 -> Sum6/2
  Sum5/1 -> P3/2
  2/1 -> Sum5/2
  P4/1 -> Sum5/1
  Sum6/1 -> P4/1
  T7/1 -> P4/2
  A1/1 -> DT1/1
  <-op5/1 -> A1/2
  T6/1 -> <-op5/2
  <-op4/1 -> A1/1
  T5/1 -> <-op4/2
  Sum2/1 -> P1/2
  1/1 -> Sum2/2
  P2/1 -> Sum2/1
  P1/1 -> Sum1/2
  In1/1 -> P/1, <-op1/1, Sum6/1, <-op5/1, <-op4/1, Sum3/1, <-op3/1, <-op2/1
  Sum3/1 -> P2/1
  T4/1 -> P2/2
  A/1 -> DT/1
  <-op3/1 -> A/2
  T3/1 -> <-op3/2
  <-op2/1 -> A/1
  T2/1 -> <-op2/2
  P/1 -> Sum1/1
  <-op1/1 -> P/2
  T1/1 -> <-op1/2
  DT/1 -> P1/1
  DT1/1 -> P3/1
  T9/1 -> P/3
  T10/1 -> Sum3/2

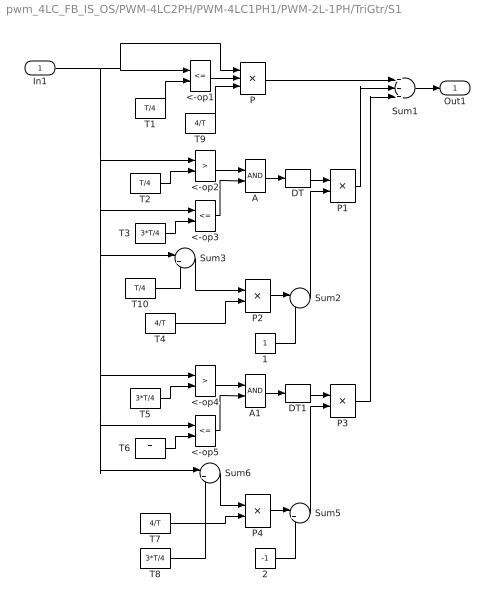
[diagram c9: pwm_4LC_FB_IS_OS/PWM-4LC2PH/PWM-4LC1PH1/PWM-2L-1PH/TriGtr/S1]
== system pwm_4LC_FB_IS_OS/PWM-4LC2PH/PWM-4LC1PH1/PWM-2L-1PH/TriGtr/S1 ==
  In1 : Inport  OutDataType=sfix(16)  OutScaling=2^0
  1 : Constant  OutDataType=sfix(16)  OutScaling=2^0
  2 : Constant  Value=-1  OutDataType=sfix(16)  OutScaling=2^0
  <-op1 : RelationalOperator  Operator=<=
  <-op2 : RelationalOperator  Operator=>
  <-op3 : RelationalOperator  Operator=<=
  <-op4 : RelationalOperator  Operator=>
  <-op5 : RelationalOperator  Operator=<=
  A : Logic  AllPortsSameDT=off
  A1 : Logic  AllPortsSameDT=off
  DT : DataTypeConversion
  DT1 : DataTypeConversion
  P : Product  Inputs=3  OutDataType=sfix(16)  OutScaling=2^0
  P{1..4} (4 alike) : Product  OutDataType=sfix(16)  OutScaling=2^0
  Sum1 : Sum  Inputs=+++  OutDataType=sfix(16)  OutScaling=2^0
  Sum2 : Sum  Inputs=|-+  OutDataType=sfix(16)  OutScaling=2^0
  Sum3 : Sum  Inputs=|+-  OutDataType=sfix(16)  OutScaling=2^0
  Sum5 : Sum  Inputs=|++  OutDataType=sfix(16)  OutScaling=2^0
  Sum6 : Sum  Inputs=|+-  OutDataType=sfix(16)  OutScaling=2^0
  T1 : Constant  Value=T/4  OutDataType=sfix(16)  OutScaling=2^0
  T10 : Constant  Value=T/4  OutDataType=sfix(16)  OutScaling=2^0
  T2 : Constant  Value=T/4  OutDataType=sfix(16)  OutScaling=2^0
  T3 : Constant  Value=3*T/4  OutDataType=sfix(16)  OutScaling=2^0
  T4 : Constant  Value=4/T  OutDataType=sfix(16)  OutScaling=2^0
  T5 : Constant  Value=3*T/4  OutDataType=sfix(16)  OutScaling=2^0
  T6 : Constant  Value=T  OutDataType=sfix(16)  OutScaling=2^0
  T7 : Constant  Value=4/T  OutDataType=sfix(16)  OutScaling=2^0
  T8 : Constant  Value=3*T/4  OutDataType=sfix(16)  OutScaling=2^0
  T9 : Constant  Value=4/T  OutDataType=sfix(16)  OutScaling=2^0
  Out1 : Outport
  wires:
  T10/1 -> Sum3/2
  T9/1 -> P/3
  DT1/1 -> P3/1
  DT/1 -> P1/1
  T1/1 -> <-op1/2
  <-op1/1 -> P/2
  P/1 -> Sum1/1
  T2/1 -> <-op2/2
  <-op2/1 -> A/1
  T3/1 -> <-op3/2
  <-op3/1 -> A/2
  A/1 -> DT/1
  T4/1 -> P2/2
  Sum3/1 -> P2/1
  In1/1 -> <-op2/1, <-op3/1, Sum3/1, <-op4/1, <-op5/1, Sum6/1, <-op1/1, P/1
  P1/1 -> Sum1/2
  P2/1 -> Sum2/1
  1/1 -> Sum2/2
  Sum2/1 -> P1/2
  T5/1 -> <-op4/2
  <-op4/1 -> A1/1
  T6/1 -> <-op5/2
  <-op5/1 -> A1/2
  A1/1 -> DT1/1
  T7/1 -> P4/2
  Sum6/1 -> P4/1
  P4/1 -> Sum5/1
  2/1 -> Sum5/2
  Sum5/1 -> P3/2
  T8/1 -> Sum6/2
  P3/1 -> Sum1/3
  Sum1/1 -> Out1/1

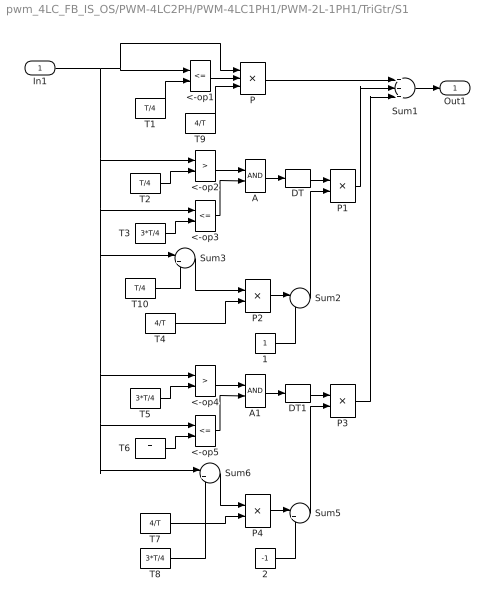
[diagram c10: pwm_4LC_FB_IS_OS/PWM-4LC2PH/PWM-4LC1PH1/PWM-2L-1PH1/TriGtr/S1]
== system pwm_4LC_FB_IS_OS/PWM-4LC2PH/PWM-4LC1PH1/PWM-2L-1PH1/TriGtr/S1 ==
  In1 : Inport  OutDataType=sfix(16)  OutScaling=2^0
  1 : Constant  OutDataType=sfix(16)  OutScaling=2^0
  2 : Constant  Value=-1  OutDataType=sfix(16)  OutScaling=2^0
  <-op1 : RelationalOperator  Operator=<=
  <-op2 : RelationalOperator  Operator=>
  <-op3 : RelationalOperator  Operator=<=
  <-op4 : RelationalOperator  Operator=>
  <-op5 : RelationalOperator  Operator=<=
  A : Logic  AllPortsSameDT=off
  A1 : Logic  AllPortsSameDT=off
  DT : DataTypeConversion
  DT1 : DataTypeConversion
  P : Product  Inputs=3  OutDataType=sfix(16)  OutScaling=2^0
  P{1..4} (4 alike) : Product  OutDataType=sfix(16)  OutScaling=2^0
  Sum1 : Sum  Inputs=+++  OutDataType=sfix(16)  OutScaling=2^0
  Sum2 : Sum  Inputs=|-+  OutDataType=sfix(16)  OutScaling=2^0
  Sum3 : Sum  Inputs=|+-  OutDataType=sfix(16)  OutScaling=2^0
  Sum5 : Sum  Inputs=|++  OutDataType=sfix(16)  OutScaling=2^0
  Sum6 : Sum  Inputs=|+-  OutDataType=sfix(16)  OutScaling=2^0
  T1 : Constant  Value=T/4  OutDataType=sfix(16)  OutScaling=2^0
  T10 : Constant  Value=T/4  OutDataType=sfix(16)  OutScaling=2^0
  T2 : Constant  Value=T/4  OutDataType=sfix(16)  OutScaling=2^0
  T3 : Constant  Value=3*T/4  OutDataType=sfix(16)  OutScaling=2^0
  T4 : Constant  Value=4/T  OutDataType=sfix(16)  OutScaling=2^0
  T5 : Constant  Value=3*T/4  OutDataType=sfix(16)  OutScaling=2^0
  T6 : Constant  Value=T  OutDataType=sfix(16)  OutScaling=2^0
  T7 : Constant  Value=4/T  OutDataType=sfix(16)  OutScaling=2^0
  T8 : Constant  Value=3*T/4  OutDataType=sfix(16)  OutScaling=2^0
  T9 : Constant  Value=4/T  OutDataType=sfix(16)  OutScaling=2^0
  Out1 : Outport
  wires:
  Sum1/1 -> Out1/1
  P3/1 -> Sum1/3
  T8/1 -> Sum6/2
  Sum5/1 -> P3/2
  2/1 -> Sum5/2
  P4/1 -> Sum5/1
  Sum6/1 -> P4/1
  T7/1 -> P4/2
  A1/1 -> DT1/1
  <-op5/1 -> A1/2
  T6/1 -> <-op5/2
  <-op4/1 -> A1/1
  T5/1 -> <-op4/2
  Sum2/1 -> P1/2
  1/1 -> Sum2/2
  P2/1 -> Sum2/1
  P1/1 -> Sum1/2
  In1/1 -> P/1, <-op1/1, Sum6/1, <-op5/1, <-op4/1, Sum3/1, <-op3/1, <-op2/1
  Sum3/1 -> P2/1
  T4/1 -> P2/2
  A/1 -> DT/1
  <-op3/1 -> A/2
  T3/1 -> <-op3/2
  <-op2/1 -> A/1
  T2/1 -> <-op2/2
  P/1 -> Sum1/1
  <-op1/1 -> P/2
  T1/1 -> <-op1/2
  DT/1 -> P1/1
  DT1/1 -> P3/1
  T9/1 -> P/3
  T10/1 -> Sum3/2

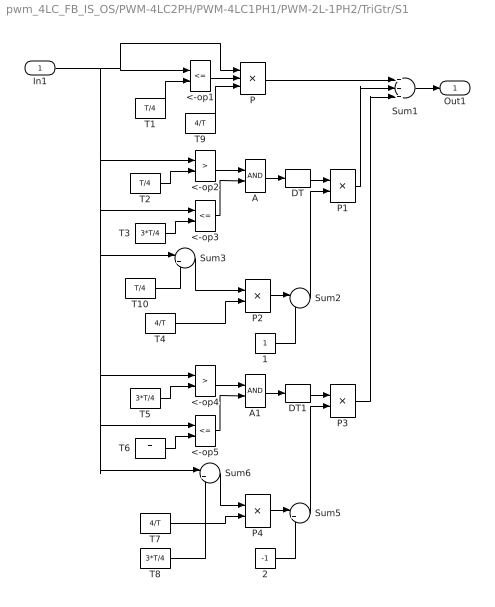
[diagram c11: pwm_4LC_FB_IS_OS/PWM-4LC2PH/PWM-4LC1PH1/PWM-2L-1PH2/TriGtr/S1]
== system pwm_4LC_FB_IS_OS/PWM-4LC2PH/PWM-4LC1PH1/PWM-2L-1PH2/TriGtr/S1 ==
  In1 : Inport  OutDataType=sfix(16)  OutScaling=2^0
  1 : Constant  OutDataType=sfix(16)  OutScaling=2^0
  2 : Constant  Value=-1  OutDataType=sfix(16)  OutScaling=2^0
  <-op1 : RelationalOperator  Operator=<=
  <-op2 : RelationalOperator  Operator=>
  <-op3 : RelationalOperator  Operator=<=
  <-op4 : RelationalOperator  Operator=>
  <-op5 : RelationalOperator  Operator=<=
  A : Logic  AllPortsSameDT=off
  A1 : Logic  AllPortsSameDT=off
  DT : DataTypeConversion
  DT1 : DataTypeConversion
  P : Product  Inputs=3  OutDataType=sfix(16)  OutScaling=2^0
  P{1..4} (4 alike) : Product  OutDataType=sfix(16)  OutScaling=2^0
  Sum1 : Sum  Inputs=+++  OutDataType=sfix(16)  OutScaling=2^0
  Sum2 : Sum  Inputs=|-+  OutDataType=sfix(16)  OutScaling=2^0
  Sum3 : Sum  Inputs=|+-  OutDataType=sfix(16)  OutScaling=2^0
  Sum5 : Sum  Inputs=|++  OutDataType=sfix(16)  OutScaling=2^0
  Sum6 : Sum  Inputs=|+-  OutDataType=sfix(16)  OutScaling=2^0
  T1 : Constant  Value=T/4  OutDataType=sfix(16)  OutScaling=2^0
  T10 : Constant  Value=T/4  OutDataType=sfix(16)  OutScaling=2^0
  T2 : Constant  Value=T/4  OutDataType=sfix(16)  OutScaling=2^0
  T3 : Constant  Value=3*T/4  OutDataType=sfix(16)  OutScaling=2^0
  T4 : Constant  Value=4/T  OutDataType=sfix(16)  OutScaling=2^0
  T5 : Constant  Value=3*T/4  OutDataType=sfix(16)  OutScaling=2^0
  T6 : Constant  Value=T  OutDataType=sfix(16)  OutScaling=2^0
  T7 : Constant  Value=4/T  OutDataType=sfix(16)  OutScaling=2^0
  T8 : Constant  Value=3*T/4  OutDataType=sfix(16)  OutScaling=2^0
  T9 : Constant  Value=4/T  OutDataType=sfix(16)  OutScaling=2^0
  Out1 : Outport
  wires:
  T10/1 -> Sum3/2
  T9/1 -> P/3
  DT1/1 -> P3/1
  DT/1 -> P1/1
  T1/1 -> <-op1/2
  <-op1/1 -> P/2
  P/1 -> Sum1/1
  T2/1 -> <-op2/2
  <-op2/1 -> A/1
  T3/1 -> <-op3/2
  <-op3/1 -> A/2
  A/1 -> DT/1
  T4/1 -> P2/2
  Sum3/1 -> P2/1
  In1/1 -> <-op2/1, <-op3/1, Sum3/1, <-op4/1, <-op5/1, Sum6/1, <-op1/1, P/1
  P1/1 -> Sum1/2
  P2/1 -> Sum2/1
  1/1 -> Sum2/2
  Sum2/1 -> P1/2
  T5/1 -> <-op4/2
  <-op4/1 -> A1/1
  T6/1 -> <-op5/2
  <-op5/1 -> A1/2
  A1/1 -> DT1/1
  T7/1 -> P4/2
  Sum6/1 -> P4/1
  P4/1 -> Sum5/1
  2/1 -> Sum5/2
  Sum5/1 -> P3/2
  T8/1 -> Sum6/2
  P3/1 -> Sum1/3
  Sum1/1 -> Out1/1
